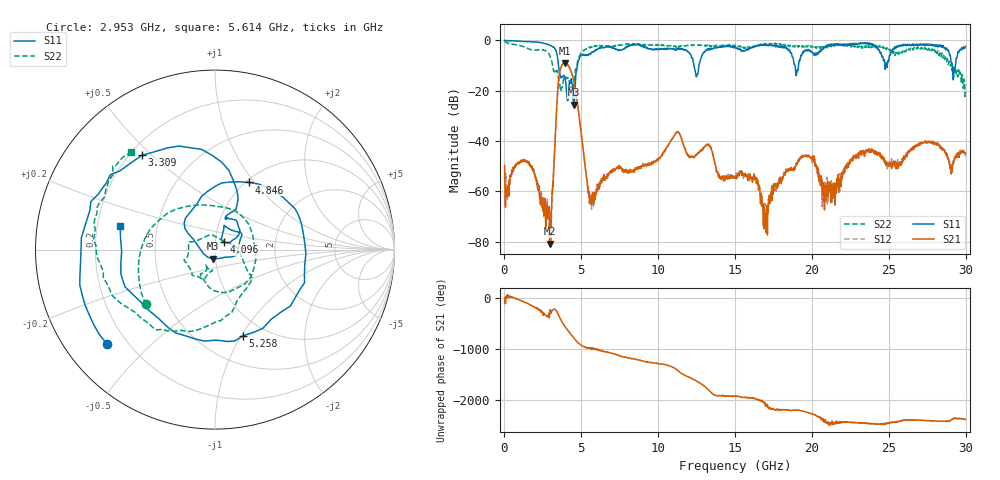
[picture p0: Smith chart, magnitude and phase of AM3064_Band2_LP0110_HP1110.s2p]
# Hz S DB R 50.0
!freq dBS11 angS11 dBS21 angS21 dBS12 angS12 dBS22 angS22
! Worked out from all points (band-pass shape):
!   1600 points, 10 MHz to 29.98 GHz, reference 50 ohm
!   highest |S21| = -9.15 dB at 3.927 GHz (marker M1); lowest = -80.8 dB at 2.934 GHz (marker M2)
!   |S21| within 3 dB of the highest: 3.609 GHz to 4.32 GHz (711.1 MHz wide, 17.9 % of centre)
!   lowest |S11| = -25.5 dB at 4.527 GHz (marker M3), VSWR 1.11, Z = 48.5 - j4.99 ohm
!   |S11| at or under -10 dB: 3.515 GHz to 4.742 GHz (1.227 GHz wide, 29.7 % of centre); 12.32 GHz to 12.65 GHz (328.1 MHz wide, 2.63 % of centre); 18.9 GHz to 19.13 GHz (228.9 MHz wide, 1.2 % of centre)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
!   |S22| runs from -23.6 to -0.3 dB; largest |S21 - S12| = 0.007
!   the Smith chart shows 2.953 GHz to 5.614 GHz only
!   S11 on the Smith chart (normalised r, x): 2.953 GHz: 0.13, -0.37; 3.309 GHz: 0.25, +0.47; 4.096 GHz: 1.10, +0.09; 4.846 GHz: 1.04, +0.94; 5.258 GHz: 0.79, -1.02; 5.614 GHz: 0.30, +0.11
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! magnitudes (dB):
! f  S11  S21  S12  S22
! 10 MHz  0.0  -49.7  -58.0  -0.3
! 1.491 GHz  -0.5  -47.9  -47.9  -3.2
! 2.934 GHz  -1.9  -80.8  -78.3  -5.9
! 2.953 GHz  -1.9  -78.5  -68.2  -6.2
! 3.309 GHz  -3.5  -37.5  -37.4  -13.1
! 3.571 GHz  -12.4  -13.2  -13.3  -16.3
! 3.927 GHz  -15.0  -9.1  -9.1  -14.9
! 4.096 GHz  -23.8  -9.8  -9.7  -15.1
! 4.527 GHz  -25.5  -16.6  -16.5  -17.3
! 4.846 GHz  -7.5  -29.6  -29.6  -6.6
! 5.015 GHz  -6.0  -38.0  -38.0  -5.0
! 5.258 GHz  -5.9  -50.6  -50.7  -3.6
! 5.614 GHz  -5.3  -63.5  -61.1  -2.9
! 10 GHz  -3.6  -46.8  -46.8  -1.9
! 11.27 GHz  -3.5  -36.2  -36.2  -2.5
! 15 GHz  -2.7  -54.2  -54.0  -2.0
! 16.35 GHz  -2.3  -54.9  -55.0  -2.4
! 16.97 GHz  -1.7  -68.8  -69.4  -1.6
! 19.99 GHz  -4.5  -46.5  -46.6  -2.3
! 20.82 GHz  -2.7  -67.3  -58.7  -2.5
! 25 GHz  -8.0  -50.1  -48.8  -3.2
! 29.98 GHz  -2.4  -44.9  -46.1  -20.3
